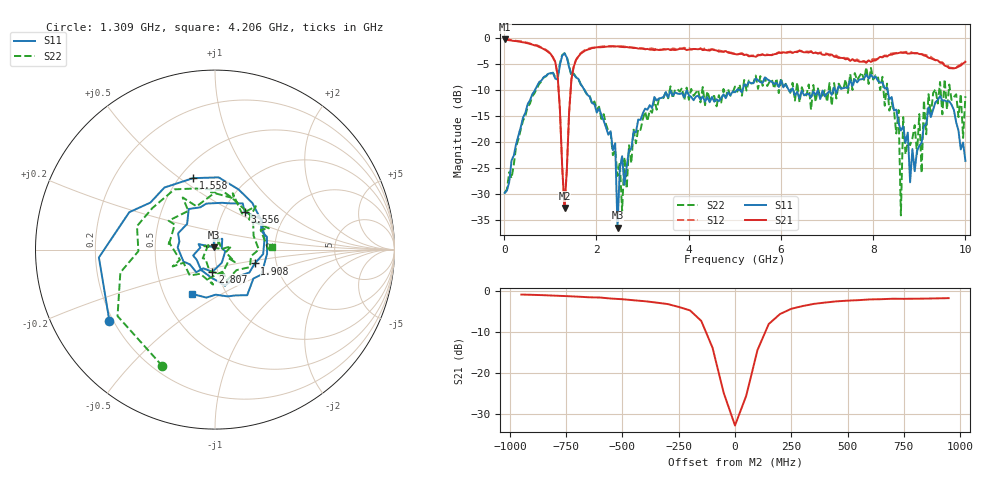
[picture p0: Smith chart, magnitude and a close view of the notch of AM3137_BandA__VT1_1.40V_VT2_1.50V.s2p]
! Date/Time: Tue, Nov 13, 2018 4:48 PM
! Network Analyzer: Agilent Technologies E8364B Rev: A.07.50.67
! Sweep from 0.010 to 10.000 GHz, 201 Points, Sweep Type: LIN
! Power Supply: 1.400 V, -0.000 A
# Hz S DB R 50
!freq MagS11 AngS11 MagS21 AngS21 MagS12 AngS12 MagS22 AngS22
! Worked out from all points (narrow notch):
!   201 points, 10 MHz to 10 GHz, reference 50 ohm
!   highest |S21| = -0.24 dB at 10 MHz (marker M1); lowest = -32.8 dB at 1.309 GHz (marker M2)
!   notch at M2: 29.9 dB deep, 166 MHz wide at half that depth
!   lowest |S11| = -36.6 dB at 2.458 GHz (marker M3), VSWR 1.03, Z = 49.3 + j1.32 ohm
!   |S11| at or under -10 dB: 1.737 GHz to 5.051 GHz (3.314 GHz wide, 97.6 % of centre); 6.265 GHz to 7.138 GHz (872.6 MHz wide, 13 % of centre); 8.311 GHz to end of sweep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
!   |S22| runs from -34.2 to -2.9 dB; largest |S21 - S12| = 0.033
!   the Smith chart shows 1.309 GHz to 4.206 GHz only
!   S11 on the Smith chart (normalised r, x): 1.309 GHz: 0.19, -0.30; 1.558 GHz: 0.58, +0.56; 1.908 GHz: 1.54, -0.25; 2.807 GHz: 0.94, -0.24; 3.556 GHz: 1.25, +0.57; 4.206 GHz: 0.69, -0.37
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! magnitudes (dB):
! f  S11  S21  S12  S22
! 10 MHz  -29.9  -0.2  -0.2  -29.9
! 1.109 GHz  -7.8  -4.6  -4.6  -7.6
! 1.309 GHz  -3.0  -32.8  -32.8  -2.9
! 1.558 GHz  -7.6  -4.3  -4.2  -7.6
! 1.708 GHz  -9.6  -2.7  -2.6  -9.5
! 1.908 GHz  -12.6  -2.0  -1.9  -12.8
! 2.408 GHz  -20.3  -1.7  -1.6  -21.5
! 2.458 GHz  -36.6  -1.6  -1.6  -26.6
! 2.807 GHz  -18.0  -1.9  -1.9  -17.7
! 3.357 GHz  -11.7  -2.3  -2.3  -11.7
! 3.556 GHz  -11.5  -2.1  -2.2  -11.6
! 4.206 GHz  -11.1  -2.2  -2.3  -10.0
! 5.005 GHz  -10.5  -3.1  -3.0  -9.4
! 6.703 GHz  -10.3  -2.9  -2.9  -9.1
! 8.352 GHz  -11.8  -3.3  -3.1  -14.0
! 8.551 GHz  -16.4  -2.9  -2.9  -13.9
! 8.601 GHz  -17.9  -2.8  -2.9  -34.2
! 8.651 GHz  -17.0  -2.9  -2.8  -15.3
! 9.001 GHz  -20.8  -3.1  -3.1  -14.7
! 9.051 GHz  -20.2  -3.1  -3.1  -26.0
! 9.101 GHz  -16.9  -3.4  -3.2  -12.0
! 10 GHz  -23.7  -4.6  -4.5  -11.2
